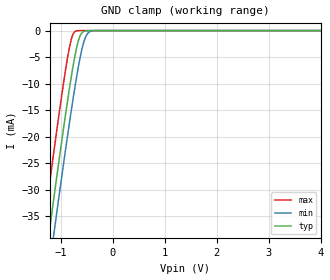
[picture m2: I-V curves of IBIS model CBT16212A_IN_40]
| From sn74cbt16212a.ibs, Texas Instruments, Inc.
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[Model]   CBT16212A_IN_40
Model_type  Input
Vinl = 0.8
Vinh = 2.0
| variable   typ   min   max
C_comp   1.31pF   1.07pF   1.68pF
[Temperature Range]   40   100   -40
| Ambient temperature   25   85   -40
[Voltage range]   4   4   4
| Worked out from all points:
|   GND clamp passes 1 mA (typ) near -0.63 V on its own axis
[GND Clamp]
| CBT16212A_IN_40
|   Voltage   I(typ)   I(min)   I(max)
-4V       -250mA     -256.3mA   -242mA
-1.365V   -48.74mA   -55.5mA    -40.02mA
-1.31V    -44.67mA   -51.45mA   -35.94mA
-1.21V    -37.33mA   -44.12mA   -28.58mA
-1.125V   -31.16mA   -37.94mA   -22.41mA
-850mV    -12.12mA   -18.65mA   -4.155mA
-780mV    -7.786mA   -14.05mA   -1.142mA
-710mV    -4.012mA   -9.712mA   -111.3uA
-630mV    -1.09mA    -5.304mA   -4.336uA
-555mV    -158.8uA   -2.167mA   -193.2nA
-405mV    -1.667uA   -91.41uA   -390.6pA
4V        28.9pA     2.697nA    22.55pA
